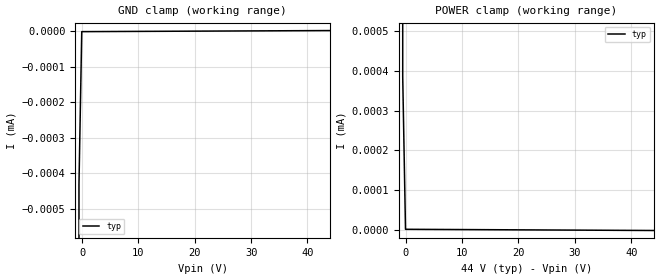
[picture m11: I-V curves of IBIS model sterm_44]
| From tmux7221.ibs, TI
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| sterm_44
[Model]   sterm_44
Model_type   Terminator
|   typ   min   max
C_comp   1.598234e-11   NA   NA
[Voltage Range]   44   NA   NA
[Temperature Range]   27   NA   NA
[Power Clamp Reference]   44   NA   NA
[GND Clamp Reference]   0   NA   NA
[GND Clamp]
|   Voltage   I(typ)   I(min)   I(max)
-5V       -4.051A    NA         NA
-1.04V    -78.38mA   NA         NA
-545.5mV  -431.2nA   NA         NA
-50.51mV  -1.525nA   NA         NA
44V       1.52nA     NA         NA
[POWER Clamp]
|   Voltage   I(typ)   I(min)   I(max)
-5V       4.768A     NA         NA
-1.04V    77.36mA    NA         NA
-545.5mV  385.6nA    NA         NA
-50.5mV   1.524nA    NA         NA
44V       -1.521nA   NA         NA
